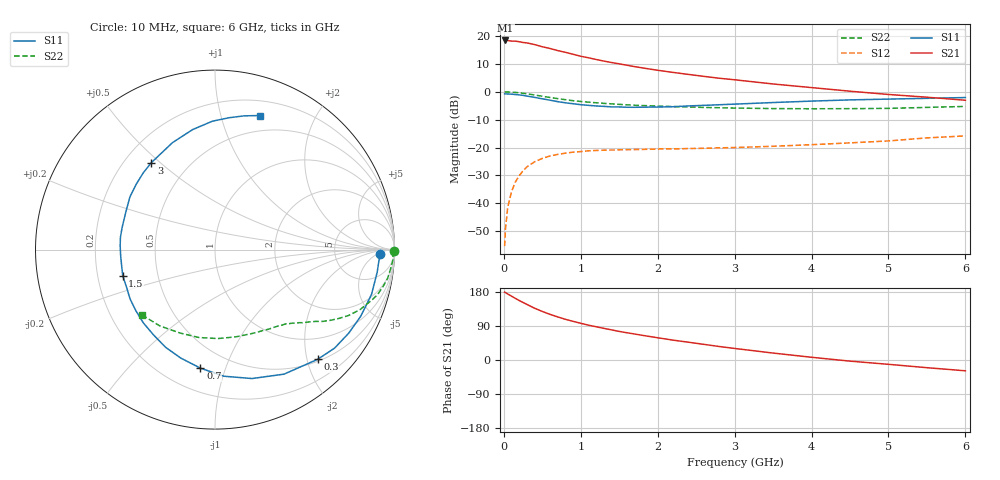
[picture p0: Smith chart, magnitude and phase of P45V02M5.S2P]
! SIEMENS Small Signal Semiconductors
! BFP182
! Si NPN RF Bipolar Junction Transistor in SOT143
! VCE = 5 V  IC = 2.5 mA
! Common Emitter S-Parameters:  March  1996
# GHz  S  MA  R  50
!  f  S11  S21  S12  S22
! GHz  MAG  ANG  MAG  ANG  MAG  ANG  MAG  ANG
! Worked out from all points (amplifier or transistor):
!   36 points, 10 MHz to 6 GHz, reference 50 ohm
!   highest |S21| = 18.4 dB at 20 MHz (marker M1)
!   |S21| within 3 dB of that: start of sweep to 616.5 MHz
!   unconditionally stable (mu >= 1): 2.074 GHz to 5.814 GHz
!   at 250 MHz: K = 0.14, MSG = 23.0 dB, |S12| = -28.3 dB
!   at 1.4 GHz: K = 0.72, MSG = 15.7 dB, |S12| = -20.9 dB
!   at 6 GHz: K = 0.97, MSG = 6.4 dB, |S12| = -15.8 dB
!   S11 on the Smith chart (normalised r, x): 10 MHz: 21, -8; 300 MHz: 0.54, -2.20; 700 MHz: 0.35, -0.82; 1.5 GHz: 0.31, -0.13; 3 GHz: 0.31, +0.47; 6 GHz: 0.34, +1.34
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0.01  0.9197 -1.7  8.195 179.0  0.0017 87.0  0.9949 -0.6
0.02  0.9165 -3.2  8.329 178.2  0.0033 95.4  0.9909 -1.2
0.05  0.9123 -8.0  8.306 174.2  0.0084 88.5  0.993 -3.2
0.15  0.8927 -24.6  8.095 162.5  0.0241 75.7  0.9748 -9.6
0.2  0.8786 -32.0  7.901 157.0  0.0313 71.8  0.9586 -12.4
0.3  0.8372 -46.9  7.532 146.8  0.045 63.9  0.9197 -17.7
0.4  0.7934 -61.0  7.025 136.6  0.0555 56.5  0.8752 -22.4
0.5  0.7473 -74.0  6.424 128.1  0.0638 50.0  0.832 -26.1
0.6  0.7072 -86.0  5.982 120.5  0.0706 45.0  0.7906 -29.0
0.7  0.6655 -97.0  5.483 113.7  0.0753 40.9  0.754 -31.5
0.8  0.6338 -107.5  5.104 107.4  0.0792 37.0  0.7211 -33.7
0.9  0.6102 -116.7  4.707 102.0  0.0826 33.9  0.6921 -35.3
1.1  0.5708 -134.5  4.073 91.9  0.0872 29.0  0.6511 -38.4
1.3  0.5473 -149.8  3.553 83.5  0.0895 25.2  0.6195 -41.1
1.5  0.5343 -164.2  3.169 75.4  0.091 22.9  0.5944 -43.6
1.8  0.5288 177.6  2.686 65.1  0.0925 20.9  0.5667 -47.4
2.2  0.5389 157.3  2.225 52.4  0.0944 19.2  0.5427 -53.1
3  0.6004 126.2  1.642 30.5  0.1001 18.9  0.5102 -66.7
3.5  0.6412 111.7  1.38 18.3  0.1052 19.2  0.4997 -76.7
4.5  0.7154 91.2  1.024 -3.0  0.1212 19.4  0.498 -100.3
5.5  0.7627 77.7  0.799 -20.3  0.1489 18.4  0.5246 -125.8
6  0.7882 71.4  0.705 -28.5  0.1616 15.1  0.5463 -138.3
